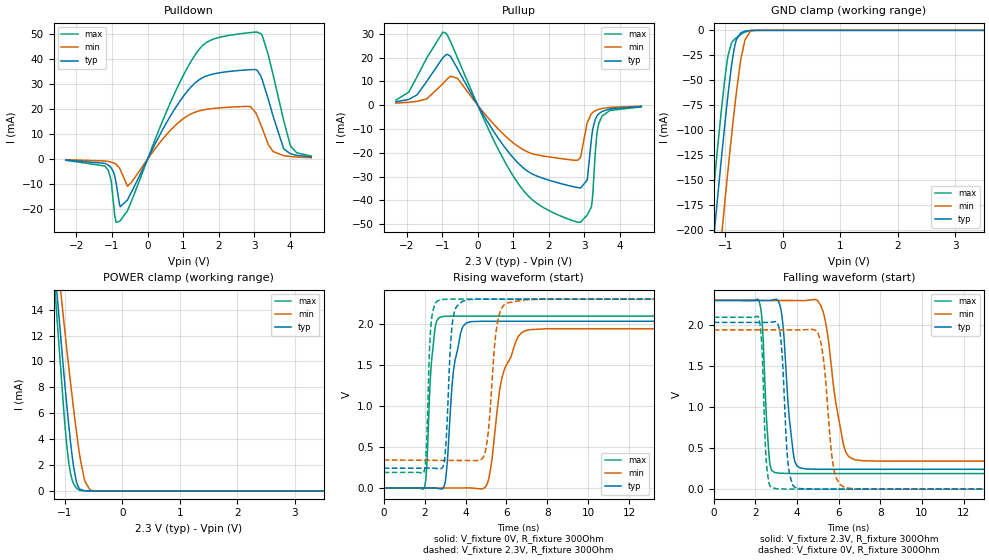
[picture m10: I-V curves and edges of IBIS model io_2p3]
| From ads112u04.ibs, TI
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|   io_2p3 Model
[Model]   io_2p3
Model_type   I/O
Polarity   Non-Inverting
Enable   Active-Low
Vinl = 0.69
Vinh = 1.61
Vmeas = 1.15
Vref = 0
Cref = 2pF
Rref = 100000
|   typ   min   max
C_comp   1.51231E-12   1.50539E-12   1.52623E-12
|C_comp_pullup   1.39199E-12   1.39197E-12   1.39841E-12
|C_comp_pulldown   1.26958E-12   1.22359E-12   1.35377E-12
[Model spec]
|subparameter
Vinl   0.69   0.6897   0.6903
Vinh   1.61   1.6093   1.6107
| Where Nom  PVT is Nominal Process, 2.3V, 27C
|   Fast PVT is Strong Process,  2.301V, -40C
|   Slow PVT is Weak Process,   2.299, 125C
[Voltage Range]   2.3   2.299   2.301
[Temperature Range]   27   125   -40
[Pullup Reference]   2.3   2.299   2.301
[Pulldown Reference]   0   0   -0
[Power Clamp Reference]   2.3   2.299   2.301
[GND Clamp Reference]   0   0   0
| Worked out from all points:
|   slope of the pulldown table from 0 to 0.345 V, typ, clamps not added: 35.7 ohm
|   slope of the pullup table from 0 to 0.345 V, typ, clamps not added: 40.1 ohm
|   GND clamp passes 1 mA (typ) near -0.67 V on its own axis
|   POWER clamp passes 1 mA (typ) near -0.81 V on its own axis
|   falling waveform, V_fixture 2.3V, R_fixture 300Ohm: 20-80 % time 361ps typ, 640ps min, 237ps max; typ from 2.3 V to 0.241 V
|   rising waveform, V_fixture 0V, R_fixture 300Ohm: 20-80 % time 420ps typ, 812ps min, 259ps max; typ from 0 V to 2.03 V
|   rising waveform, V_fixture 2.3V, R_fixture 300Ohm: 20-80 % time 239ps typ, 366ps min, 171ps max; typ from 0.241 V to 2.3 V
|   falling waveform, V_fixture 0V, R_fixture 300Ohm: 20-80 % time 247ps typ, 398ps min, 179ps max; typ from 2.03 V to 0 V
[Pulldown]
|   Voltage   I(typ)   I(min)   I(max)
-2.3V     -376.1uA   -210.5uA   -461uA
-1.196V   -1.735mA   -769.4uA   -2.834mA
-1.03V    -3.336mA   -1.185mA   -8.215mA
-954.5mV  -5.328mA   -1.543mA   -18.13mA
-788.9mV  -18.21mA   -3.605mA   -24.81mA
-568.1mV  -16.33mA   -10.78mA   -20.62mA
1.371V    30.78mA    18.88mA    42.25mA
3.041V    35.64mA    18.46mA    50.6mA
3.386V    24.15mA    6.086mA    41.84mA
3.827V    4.055mA    1.361mA    15.31mA
4.02V     2.11mA     1.007mA    5.15mA
4.6V      908.2uA    565.3uA    1.225mA
[GND Clamp]
|   Voltage   I(typ)   I(min)   I(max)
-2.3V     -915.1mA   -992.7mA   -866.9mA
-1.389V   -326mA     -406.1mA   -275.6mA
-1.161V   -184.4mA   -264.3mA   -134.3mA
-1.079V   -134.9mA   -214.1mA   -86.07mA
-1.017V   -99.16mA   -177.1mA   -52.96mA
-947.6mV  -62.02mA   -137.2mA   -24.1mA
-892.4mV  -35.98mA   -106.4mA   -12.94mA
-830.3mV  -14.51mA   -73.77mA   -8.554mA
-726.8mV  -2.444mA   -28.28mA   -3.999mA
-657.8mV  -829.5uA   -9.725mA   -1.774mA
-492.2mV  -20.78uA   -199.7uA   -37.46uA
4.6V      0A         0A         0A
[Pullup]
|   Voltage   I(typ)   I(min)   I(max)
-2.3V     1.451mA    876.4uA    2.144mA
-1.707V   4.343mA    1.629mA    11.97mA
-885.5mV  21.27mA    10.62mA    30.22mA
-568.1mV  15.34mA    11.32mA    19.89mA
418.6mV   -10.33mA   -7.477mA   -13.75mA
1.171V    -24.86mA   -17.71mA   -33.66mA
2.82V     -34.68mA   -23.03mA   -49.21mA
3.075V    -31.53mA   -7.523mA   -46.24mA
3.192V    -14.79mA   -3.696mA   -42.87mA
3.344V    -4.808mA   -2.045mA   -12.83mA
3.496V    -2.603mA   -1.371mA   -4.542mA
4.6V      -539.4uA   -366uA     -683.9uA
[POWER Clamp]
|   Voltage   I(typ)   I(min)   I(max)
-2.3V     81.56mA    72.07mA    93.62mA
-1.217V   19.41mA    21.52mA    18.32mA
-1.161V   16.42mA    19.1mA     14.71mA
-1.148V   15.67mA    18.5mA     13.82mA
-1.017V   8.898mA    12.93mA    5.906mA
-940.7mV  5.333mA    9.829mA    2.393mA
-906.2mV  3.867mA    8.461mA    1.399mA
-851mV    1.877mA    6.351mA    565.9uA
-768.2mV  301.1uA    3.474mA    96.12uA
-657.8mV  12.92uA    780.8uA    3.79uA
-519.8mV  251.8nA    24.93uA    20.6nA
4.6V      0A         0A         0A
[Ramp]
R_load = 300
|   typ   min   max
dV/dt_r   1.21887/4.20021e-10   1.16426/8.23436e-10   1.25651/2.59394e-10
dV/dt_f   1.23544/3.61413e-10   1.17475/6.42013e-10   1.26664/2.36341e-10
[Falling Waveform]
V_fixture = 2.3V
V_fixture_min = 2.299V
V_fixture_max = 2.301V
R_fixture = 300Ohm
C_fixture = 0F
|   Time   V(typ)   V(min)   V(max)
0s        2.3V       2.299V     2.301V
2.161ns   2.299V     2.298V     2.301V
2.684ns   2.299V     2.298V     335.9mV
3.141ns   2.267V     2.298V     194.3mV
3.808ns   465mV      2.298V     190.5mV
4.153ns   257.7mV    2.298V     190.5mV
5.23ns    241.8mV    2.181V     190.5mV
6.208ns   241.8mV    574.7mV    190.5mV
6.752ns   241.8mV    360.6mV    190.5mV
50ns      240.9mV    341.1mV    189.9mV
[Rising Waveform]
V_fixture = 0V
V_fixture_min = 0V
V_fixture_max = 0V
R_fixture = 300Ohm
C_fixture = 0F
|   Time   V(typ)   V(min)   V(max)
0s        -91.48nV   978.7pV    -348.3nV
1.975ns   624.4uV    295.8uV    -161.5uV
2.48ns    783.9uV    371.3uV    1.884V
2.903ns   -693.8uV   434.7uV    2.09V
3.488ns   1.555V     522.3uV    2.094V
4.277ns   2.026V     318.2uV    2.094V
5.089ns   2.031V     72.16mV    2.094V
5.779ns   2.031V     1.342V     2.094V
7.102ns   2.031V     1.928V     2.094V
50ns      2.031V     1.94V      2.094V
[Rising Waveform]
V_fixture = 2.3V
V_fixture_min = 2.299V
V_fixture_max = 2.301V
R_fixture = 300Ohm
C_fixture = 0F
|   Time   V(typ)   V(min)   V(max)
0s        240.9mV    341.1mV    189.9mV
1.961ns   241.2mV    338mV      190.7mV
2.323ns   241.3mV    337.5mV    2.016V
2.792ns   236mV      336.7mV    2.295V
3.372ns   2.037V     335.8mV    2.301V
4.097ns   2.294V     334.7mV    2.301V
4.978ns   2.299V     455.6mV    2.301V
5.691ns   2.299V     2.149V     2.301V
6.887ns   2.299V     2.291V     2.301V
50ns      2.3V       2.299V     2.301V
[Falling Waveform]
|Gnd
V_fixture = 0V
V_fixture_min = 0V
V_fixture_max = 0V
R_fixture = 300Ohm
C_fixture = 0F
|   Time   V(typ)   V(min)   V(max)
0s        2.031V     1.94V      2.094V
2.146ns   2.031V     1.94V      2.096V
2.55ns    2.031V     1.94V      265.5mV
3.052ns   2.027V     1.94V      4.677mV
3.604ns   240.3mV    1.94V      628.6uV
4.202ns   5.888mV    1.94V      628.2uV
5.115ns   817.1uV    1.819V     627.7uV
5.749ns   816.6uV    271.4mV    627.3uV
6.28ns    816.1uV    21.16mV    626.9uV
50ns      -61.67nV   1.151nV    -382nV
